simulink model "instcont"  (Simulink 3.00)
settings: Solver=ode45  StartTime=0.0  StopTime=2  MaxStep=1  RelTol=1e-3  AbsTol=1e-3
undefined symbols (not defined in the file or in its folder): sfunyst

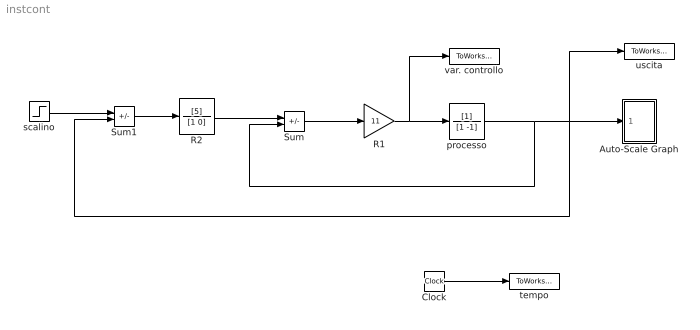
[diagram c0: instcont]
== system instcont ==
  Auto-Scale Graph : Subsystem  mask(Storage scope.){}
      mask help: Storage scope using MATLAB graph window. Enter plotting ranges and line type.
      mask init:
      | npts = @4; color = @5; ax = [0, @1, @2, @3]; dt=-1;
  Clock : Clock
  R1 : Gain  Gain=11  SaturateOnIntegerOverflow=on
  R2 : TransferFcn  Numerator=[5]  Denominator=[1 0]
  Sum : Sum  Inputs=+-  SaturateOnIntegerOverflow=on
  Sum1 : Sum  Inputs=+-  SaturateOnIntegerOverflow=on
  processo : TransferFcn  Numerator=[1]  Denominator=[1 -1]
  scalino : Step  Time=0  Before=0  After=1  SampleTime=1
  tempo : ToWorkspace  VariableName=t  SampleTime=0  SaveFormat=Matrix
  uscita : ToWorkspace  VariableName=y  SampleTime=0  SaveFormat=Matrix
  var. controllo : ToWorkspace  VariableName=u  SampleTime=0  SaveFormat=Matrix
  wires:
  Sum/1 -> R1/1
  Sum1/1 -> R2/1
  processo/1 -> Sum/2, Auto-Scale Graph/1(x), Sum1/2, uscita/1
  scalino/1 -> Sum1/1
  R2/1 -> Sum/1
  Clock/1 -> tempo/1
  R1/1 -> processo/1, var. controllo/1

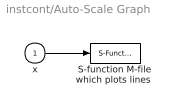
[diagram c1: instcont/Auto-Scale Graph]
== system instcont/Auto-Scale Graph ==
  x : Inport  Port=1  PortWidth=-1  SampleTime=-1  DataType=auto
  "S-function M-file which plots lines " : S-Function  LoadFcn=sfunyst([],[],[],'LoadBlock')  FunctionName=sfunyst  Parameters=ax, color, npts, dt  PortCounts=[]  SFunctionModules=''
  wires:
  x/1 -> "S-function M-file which plots lines "/1
